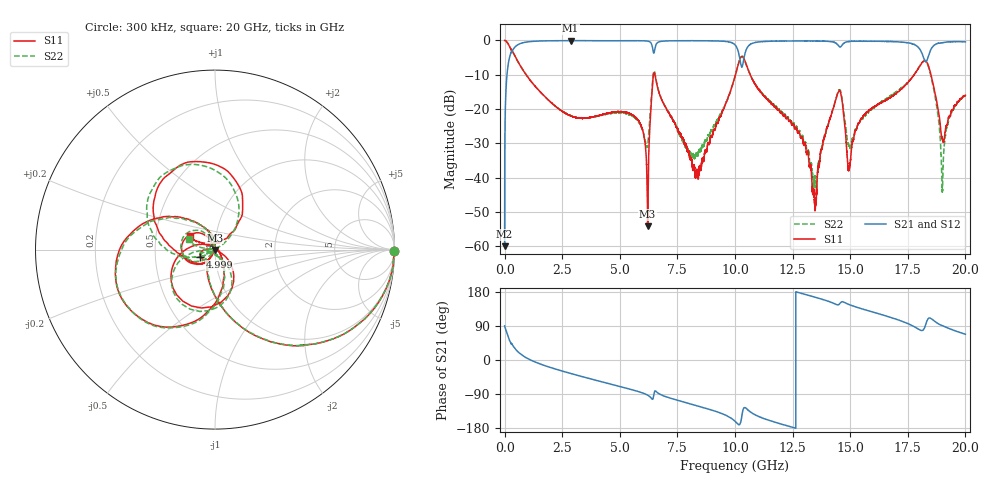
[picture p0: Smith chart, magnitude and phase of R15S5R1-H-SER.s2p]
!{R15S5R1}
!Johanson Technology Inc.
!www.johansontechnology.com
!Test Board Conditions:
!Substrate Type  RO4350B
!Substrate Thickness  20 mil
!Substrate Dk  3.66
!TL Type: GCPW
!TL Trace Width  34 mil
!TL Gap  10 mil
!Electrode orientation  Horizontal
!DUT TOPOLOGY	SERIES
!Mounting Pad LxW  26x52 mil
! Created Sat Feb  6 13:58:20 2021
# hz S ma R 50
! 2 Port Network Data from SP1.SP block
! freq  magS11  angS11  magS21  angS21  magS12  angS12  magS22  angS22
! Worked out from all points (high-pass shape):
!   20001 points, 300 kHz to 20 GHz, reference 50 ohm
!   highest |S21| = -0.05 dB at 2.861 GHz (marker M1); lowest = -60.0 dB at 300 kHz (marker M2)
!   |S21| within 3 dB of the highest: 334 MHz to 6.445 GHz (6.111 GHz wide, 180 % of centre); 10.47 GHz to 18.06 GHz (7.595 GHz wide, 53.2 % of centre)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
!   lowest |S11| = -54.2 dB at 6.208 GHz (marker M3), VSWR 1.00, Z = 49.9 - j0.17 ohm
!   |S11| at or under -10 dB: 934.2 MHz to 6.46 GHz (5.526 GHz wide, 149 % of centre); 6.527 GHz to 10.02 GHz (3.494 GHz wide, 42.2 % of centre); 10.66 GHz to 17.77 GHz (7.115 GHz wide, 50 % of centre)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
!   |S22| runs from -44.3 to 0.0 dB; largest |S21 - S12| = 0.013
!   S11 on the Smith chart (normalised r, x): 300 kHz: open; 4.999 GHz: 0.85, -0.07; 20 GHz: 0.75, +0.12
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300000  0.9998 -0.4  0.001003 90.1  0.001146 89.2  1 -0.3
1.133e8  0.9378 -21.8  0.3429 68.0  0.3439 68.0  0.9374 -21.7
3.143e8  0.7262 -47.4  0.6821 42.4  0.6836 42.5  0.7265 -47.2
1.0323e9  0.2848 -87.1  0.9549 2.9  0.9562 2.9  0.2845 -87.0
2.8613e9  0.0793 -122.6  0.9948 -35.4  0.9929 -35.4  0.08036 -126.3
3.3343e9  0.07409 -126.9  0.993 -43.2  0.9924 -43.3  0.0748 -137.4
4.9993e9  0.09161 -153.8  0.9897 -69.8  0.9903 -69.8  0.08804 -163.8
5.8633e9  0.06327 -178.3  0.9905 -84.4  0.99 -84.4  0.06145 -164.5
6.2083e9  0.001953 -119.4  0.9777 -92.7  0.9785 -92.6  0.03009 -89.9
6.4473e9  0.2932 -82.7  0.6972 -101.0  0.6974 -100.8  0.316 -85.3
6.6673e9  0.1894 -173.9  0.9447 -87.7  0.9463 -87.6  0.1944 -163.6
8.3483e9  0.01236 52.0  0.9888 -120.7  0.9913 -120.6  0.02147 -95.5
1.00003e10  0.2985 -89.8  0.8628 -161.6  0.863 -161.6  0.2986 -88.0
1.03713e10  0.5566 -172.5  0.5129 -127.7  0.5125 -127.8  0.5564 -170.5
1.33343e10  0.009149 108.0  0.9822 168.2  0.9832 168.2  0.01444 113.0
1.34693e10  0.003809 -152.0  0.9824 165.8  0.9813 165.8  0.009787 163.0
1.44913e10  0.1798 -169.1  0.8379 145.8  0.8407 145.9  0.1863 -177.1
1.49483e10  0.01298 -166.3  0.9667 146.5  0.9647 146.6  0.02919 156.9
1.66673e10  0.1436 -152.0  0.9686 114.0  0.9591 113.9  0.1496 -163.5
1.82873e10  0.4978 100.1  0.4893 95.2  0.488 95.6  0.4962 106.7
1.90123e10  0.03548 93.3  0.9272 90.4  0.9236 90.3  0.008403 140.0
2e10  0.1597 151.8  0.9557 67.9  0.9499 67.5  0.1566 158.2
